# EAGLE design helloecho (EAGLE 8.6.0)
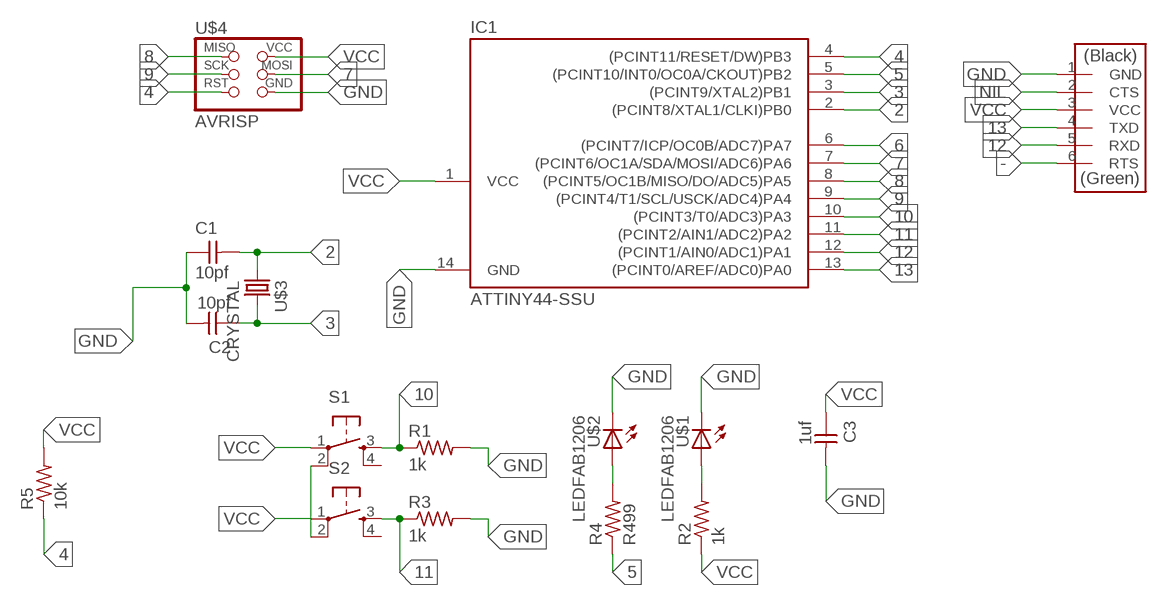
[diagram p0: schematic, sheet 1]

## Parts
C1  10pf  CAP-UNPOLARIZEDFAB  [C1206FAB]
C2  10pf  CAP-UNPOLARIZEDFAB  [C1206FAB]
C3  1uf  CAP-UNPOLARIZEDFAB  [C1206FAB]
IC1  ATTINY44-SSU  [SOIC14]
R1  1k  RES-US1206  [R1206]
R2  1k  RES-US1206  [R1206]
R3  1k  RES-US1206  [R1206]
R4  R499  RES-US1206  [R1206]
R5  10k  RES-US1206FAB  [R1206FAB]
S1  6MM_SWITCH6MM_SWITCH  [6MM_SWITCH]
S2  6MM_SWITCH6MM_SWITCH  [6MM_SWITCH]
U$1  LEDFAB1206  [LED1206FAB]
U$2  LEDFAB1206  [LED1206FAB]
U$3  CRYSTAL  [2-SMD-5X3MM]
U$4  AVRISP  [2X03]
U$5  FTDI-SMD-HEADER  [1X06SMD]

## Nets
2: C1.2 IC1.2((PCINT8/XTAL1/CLKI)PB0) U$3.P$1
3: C2.1 IC1.3((PCINT9/XTAL2)PB1) U$3.P$2
4: IC1.4((PCINT11/RESET/DW)PB3) R5.1 U$4.5(RST)
5: IC1.5((PCINT10/INT0/OC0A/CKOUT)PB2) R4.1
6: IC1.6((PCINT7/ICP/OC0B/ADC7)PA7)
7: IC1.7((PCINT6/OC1A/SDA/MOSI/ADC6)PA6) U$4.4(MOSI)
8: IC1.8((PCINT5/OC1B/MISO/DO/ADC5)PA5) U$4.1(MISO)
9: IC1.9((PCINT4/T1/SCL/USCK/ADC4)PA4) U$4.3(SCK)
10: IC1.10((PCINT3/T0/ADC3)PA3) R1.1 S1.3(S)
11: IC1.11((PCINT2/AIN1/ADC2)PA2) R3.1 S2.3(S)
12: IC1.12((PCINT1/AIN0/ADC1)PA1) U$5.5(RXD)
13: IC1.13((PCINT0/AREF/ADC0)PA0) U$5.4(TXD)
-: U$5.6(RTS)
GND: C1.1 C2.2 C3.2 IC1.14(GND) R1.2 R3.2 U$1.2(C) U$2.2(C) U$4.6(GND) U$5.1(GND)
N$1: S1.2(P1) S2.2(P1)
N$10: R4.2 U$2.1(A)
N$13: R2.2 U$1.1(A)
NIL: U$5.2(CTS)
VCC: C3.1 IC1.1(VCC) R2.1 R5.2 S1.1(P) S2.1(P) U$4.2(VCC) U$5.3(VCC)
Unconnected: S1.4(S1) S2.4(S1)

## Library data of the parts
C1-C3 = fab:CAP-UNPOLARIZED
IC1 = fab:ATTINY44
R1-R5 = fab:RES-US: Resistor (US Symbol)
S1 S2 = fab:6MM_SWITCH: OMRON SWITCH
U$1 U$2 = fab:LED: LED
U$3 = fab:CRYSTAL
U$4 = fab:AVRISP
U$5 = fab:FTDI-SMD-HEADER

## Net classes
0 default: width 0.4 mm, drill 0.4 mm, clearance 0.4 mm

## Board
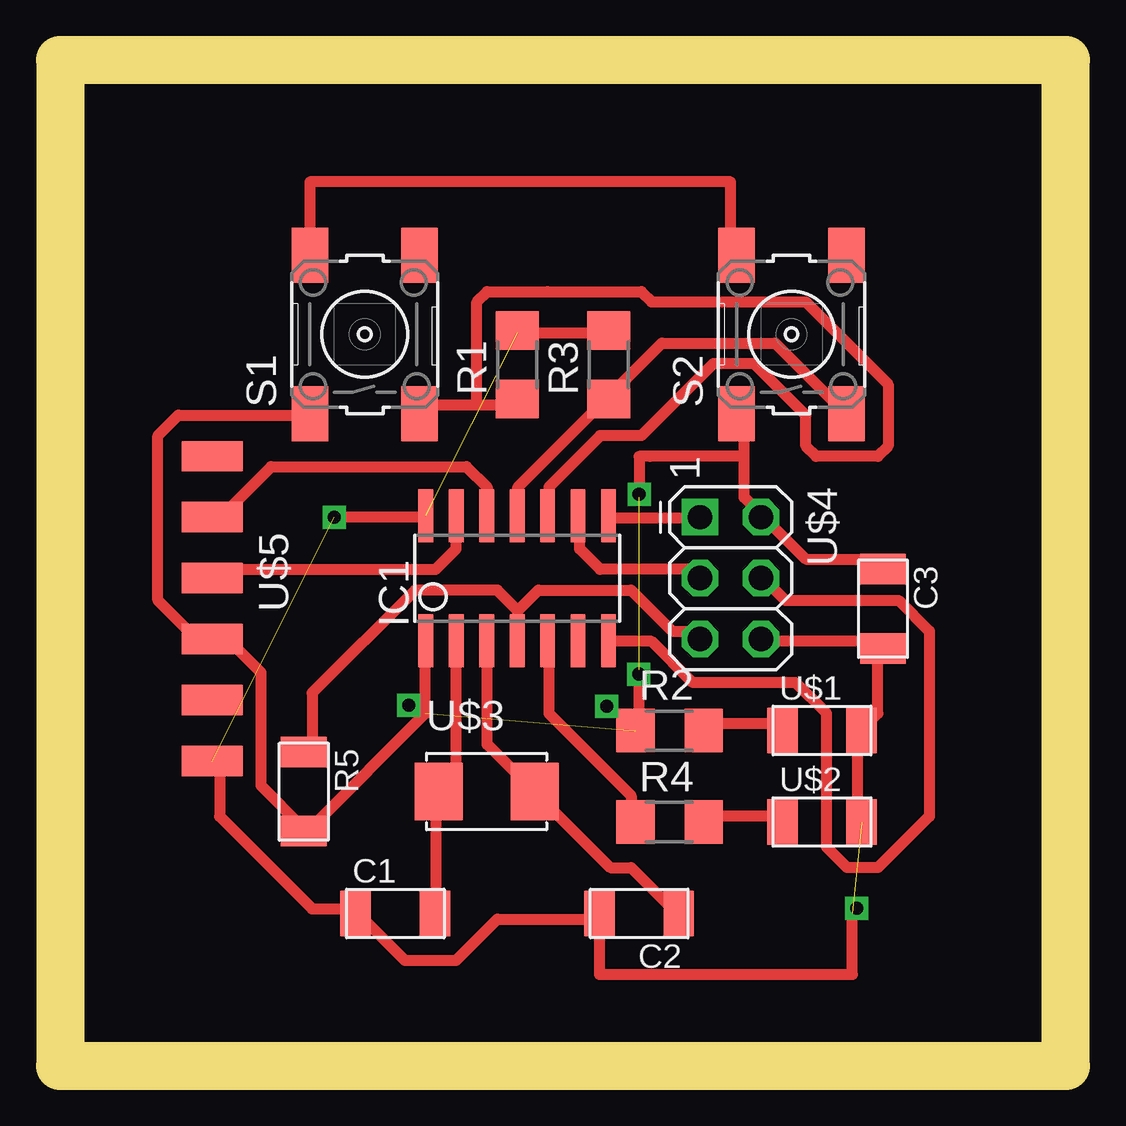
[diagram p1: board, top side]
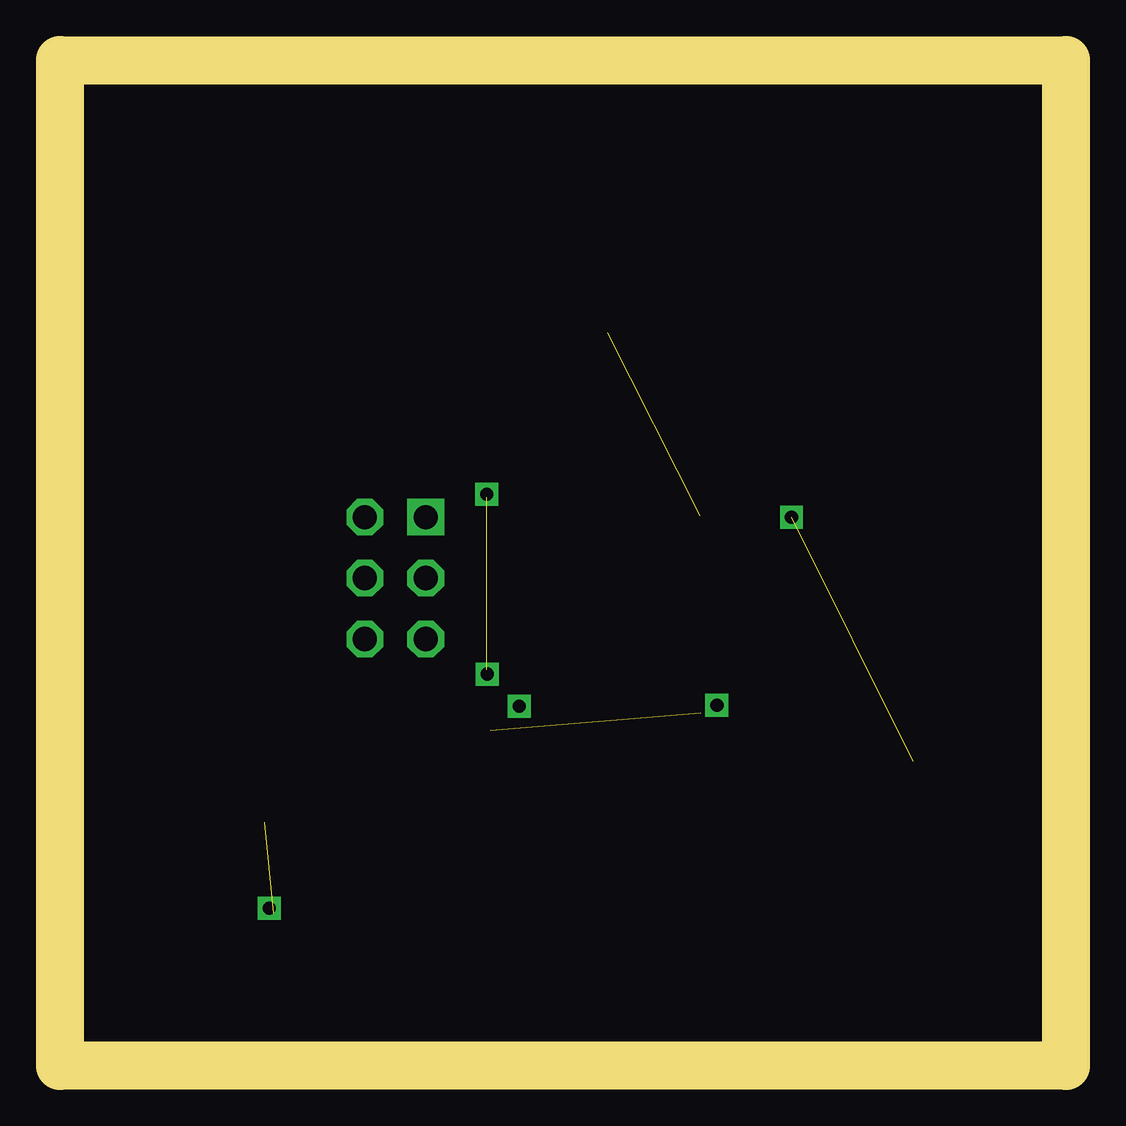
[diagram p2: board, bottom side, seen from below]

Size 41.91 x 41.91 mm. Coordinates in mm from the lower left corner, seen from the top.
Outline: 41.91,41.91 0,41.91 0,0 41.91,0 41.91,41.91
Copper layers (1*16): Top 0.035mm / dielectric 1.5mm / Bottom 0.035mm
Design rules "default *": minimum track width 18mil, minimum drill 0.35mm, track to track 12mil, track to pad 12mil, pad to pad 12mil, via to via 12mil, smd to smd 12mil, copper to edge 60mil, drill to drill 6mil, minimum pad ring 10mil, minimum via ring 8mil, stop-mask expansion 4mil, vias tented up to drill 0mil, thermal gap 10mil

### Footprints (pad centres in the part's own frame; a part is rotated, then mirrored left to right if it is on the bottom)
C1206FAB = smd 1.27 x 1.905: 1 -1.651,0; 2 1.651,0
SOIC14 = smd 0.61 x 2.21: 1 -3.81,-2.603; 2 -2.54,-2.603; 3 -1.27,-2.603; 4 0,-2.603; 5 1.27,-2.603; 6 2.54,-2.603; 7 3.81,-2.603; 8 3.81,2.603; 9 2.54,2.603; 10 1.27,2.603; 11 0,2.603; 12 -1.27,2.603; 13 -2.54,2.603; 14 -3.81,2.603
R1206 = smd 1.6 x 1.803: 1 -1.422,0; 2 1.422,0
R1206FAB = smd 1.27 x 1.905: 1 -1.651,0; 2 1.651,0
6MM_SWITCH = smd 2.286 x 1.524: 1 -3.302,2.286; 2 3.302,2.286; 3 -3.302,-2.286; 4 3.302,-2.286
LED1206FAB = smd 1.27 x 1.905: 1 -1.651,0; 2 1.651,0
2-SMD-5X3MM = smd 2 x 2.4: P$1 -2,0; P$2 2,0
2X03 = drill 1.016 square: 1 -2.54,-1.27 | drill 1.016 octagon: 2 -2.54,1.27; 3 0,-1.27; 4 0,1.27; 5 2.54,-1.27; 6 2.54,1.27
1X06SMD = smd 2.54 x 1.27: 1 0,6.35; 2 0,3.81; 3 0,1.27; 4 0,-1.27; 5 0,-3.81; 6 0,-6.35

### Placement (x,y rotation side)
C1  13.97,6.35 0 top
C2  24.13,6.35 180 top
C3  34.29,19.05 270 top
IC1  19.05,20.32 0 top
R1  19.05,29.21 90 top
R2  25.4,13.97 0 top
R3  22.86,29.21 90 top
R4  25.4,10.16 0 top
R5  10.16,11.43 270 top
S1  12.7,30.48 90 top
S2  30.48,30.48 90 top
U$1  31.75,13.97 0 top
U$2  31.75,10.16 0 top
U$3  17.78,11.43 0 top
U$4  27.94,20.32 270 top
U$5  6.35,19.05 180 top

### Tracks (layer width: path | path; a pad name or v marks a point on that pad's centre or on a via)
2
  Top 0.457: C1.2 15.65,6.54 15.65,11.25 U$3.P$1 16.08,11.68 16.51,12.11 16.51,17.68 IC1.2
3
  Top 0.457: C2.1 25.51,6.54 23.79,8.25 22.94,8.25 19.94,11.25 U$3.P$2 19.51,11.68 17.79,13.4 17.79,17.68 IC1.3
4
  Top 0.457: 19.08,18.97 18.22,19.83 14.79,19.83 10.51,15.54 10.51,13.4 R5.1 | 19.08,18.97 19.08,18.11 IC1.4 | 19.08,18.97 19.94,19.83 23.79,19.83 25.51,18.11 26.37,18.11 U$4.5
5
  Top 0.457: R4.1 23.79,10.4 23.79,11.25 20.37,14.68 20.37,17.68 IC1.5
7
  Top 0.457: IC1.7 22.94,17.68 24.65,17.68 26.37,15.97 30.65,15.97 31.94,14.68 31.94,9.11 32.8,8.25 34.08,8.25 36.22,10.4 36.22,18.11 34.94,19.4 30.22,19.4 29.37,20.25 U$4.4
8
  Top 0.457: IC1.8 22.94,22.83 26.37,22.83 U$4.1
9
  Top 0.457: IC1.9 21.65,22.83 21.65,21.54 22.51,20.68 26.37,20.68 U$4.3
10
  Top 0.457: 17.37,27.54 15.22,27.54 S1.3 | 17.37,27.54 18.65,27.54 R1.1 | 17.37,27.54 17.37,31.83 17.79,32.26 20.32,32.26 24.22,32.26 24.65,31.83 31.08,31.83 34.51,28.4 34.51,25.83 34.08,25.4 31.51,25.4 31.08,25.83 31.08,27.11 28.94,29.26 27.22,29.26 24.22,26.26 22.51,26.26 20.37,24.11 20.37,23.26 IC1.10
11
  Top 0.457: IC1.11 19.08,23.26 19.08,24.11 22.51,27.54 R3.1 22.94,27.97 25.08,30.11 29.8,30.11 32.37,27.54 S2.3
12
  Top 0.457: IC1.12 17.79,23.26 17.79,24.11 16.94,24.97 8.79,24.97 6.65,22.83 U$5.5
13
  Top 0.457: IC1.13 16.51,22.83 16.51,21.54 15.65,20.68 6.65,20.68 U$5.4
GND  (via drill 0.55)  (3 unrouted)
  Top 0.457: U$5.1 6.65,12.54 6.65,10.4 10.51,6.54 12.22,6.54 C1.1 12.65,6.11 14.37,4.4 16.51,4.4 18.22,6.11 22.08,6.11 C2.2 22.48,3.81 33.02,3.81 33.02,6.35 | R1.2 19.08,30.54 22.51,30.54 R3.2 | U$2.2 33.22,10.4 33.22,13.83 U$1.2 33.65,14.25 34.08,14.68 34.08,17.25 C3.2 34.08,17.68 29.37,17.68 U$4.6 | IC1.14 15.24,22.86 v11.43,22.86
N$1
  Top 0.457: S2.2 27.94,33.78 27.94,36.83 10.41,36.83 S1.2
N$2  (via drill 0.55)
  other vias: 24.11,16.32
N$3  (via drill 0.55)
  other vias: 24.13,23.82
N$4  (via drill 0.55)
  other vias: 14.54,15.03
N$5  (via drill 0.55)
  other vias: 22.78,14.98
N$6  (via drill 0.55)
  other vias: 33.19,6.56
N$10
  Top 0.457: R4.2 27.22,10.4 29.8,10.4 U$2.1
N$13
  Top 0.457: R2.2 27.22,14.25 29.8,14.25 U$1.1
VCC  (2 unrouted)
  Top 0.457: IC1.1 15.22,17.68 15.22,14.68 10.51,9.97 R5.2 10.08,9.97 8.36,11.68 8.36,16.4 6.65,18.11 U$5.3 6.22,18.11 5.36,18.11 4.08,19.4 4.08,26.26 4.94,27.11 10.08,27.11 S1.1 | C3.1 34.08,21.11 31.08,21.11 29.37,22.83 U$4.2 28.94,23.26 28.51,23.68 28.51,25.4 | 28.51,25.4 28.51,27.11 S2.1 | 28.51,25.4 24.58,25.4 24.13,25.4 24.13,23.68 | R2.1 24.13,13.97 24.13,16.51
(copper drawn outside any net)
  shapes: Bottom circle x6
